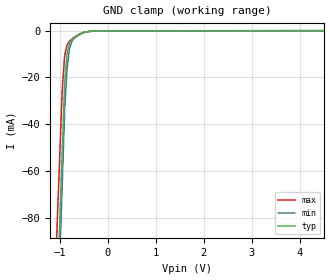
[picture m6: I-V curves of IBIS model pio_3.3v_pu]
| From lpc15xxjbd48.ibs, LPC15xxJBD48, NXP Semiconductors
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[Model] pio_3.3v_pu
Model_type Input
Vinl = 990.000mV
Vinh = 2.31000V
C_comp 598.000fF 598.000fF 598.000fF
| variable typ   min   max
[Voltage Range] 3.30000V 3.00000V 3.60000V
[POWER Clamp Reference] 3.30000V 3.00000V 3.60000V
[GND Clamp Reference] 0.00000V 0.00000V 0.00000V
[Temperature Range]   25   85   -40
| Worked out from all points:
|   GND clamp passes 1 mA (typ) near -0.53 V on its own axis
[GND Clamp]
-3.3V     -1.424A    -1.553A    -1.303A
-950mV    -51.27mA   -65.75mA   -24.89mA
-900mV    -22.07mA   -34.11mA   -10.62mA
-850mV    -9.837mA   -16.38mA   -6.087mA
-800mV    -5.504mA   -7.708mA   -4.527mA
-750mV    -3.952mA   -4.58mA    -3.621mA
-700mV    -3.012mA   -3.291mA   -2.716mA
-550mV    -1.229mA   -1.345mA   -990.9uA
-400mV    -344.5uA   -361.6uA   -322.3uA
50mV      -67.82uA   -60.48uA   -85.59uA
6.6V      38.6uA     43.62uA    40.34uA
[POWER Clamp]
-3.3V     0A         0A         0A
6.6V      0A         0A         0A
